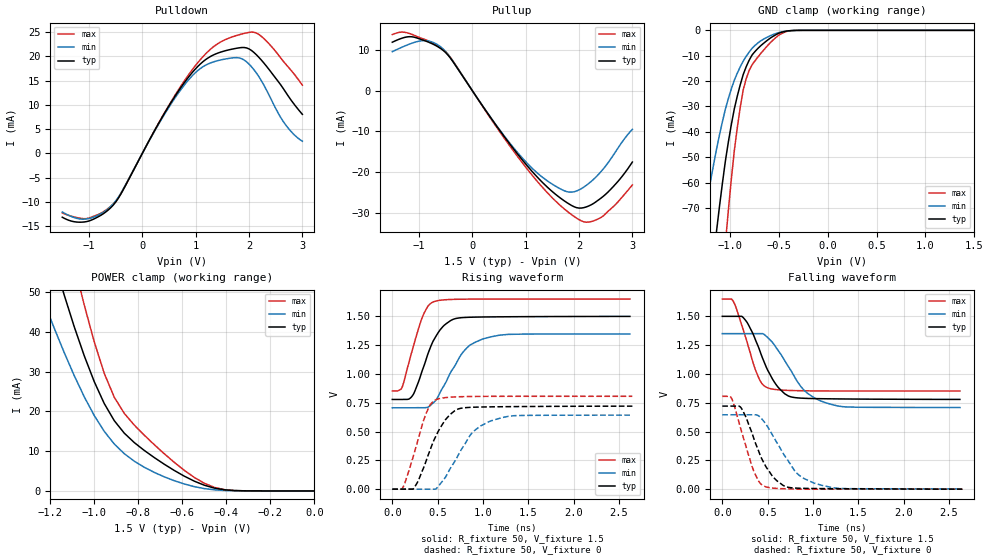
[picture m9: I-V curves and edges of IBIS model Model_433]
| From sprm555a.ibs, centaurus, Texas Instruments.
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| Model based on original model for BCSHTLTCSCDDVPBFZ_SSGFV
|   Sub model SR10_7MA_PADN_10PER_1P5
[model]   Model_433
|[Description]  [1.5V-3-STATE-X-SLOW:7MA, IND, 10%]
|   Slow slew rate (SR[1:0] = "01"), 1.14 * RExt = 0.875 * Iout
|   (I[2:0] = "010"), 7mA nominal with Rext = 50R, ,Industrial
|   temperature range (-40C to 125C, 25C nominal),10% power supply
|   tolerance
|[Input Load]
|[Output Drive] SLOW:7MA
|Voltage   1.5V
|Mode   3-STATE
Model_type   3-state
Polarity   Non-Inverting
Enable   Active-Low
Cref =  15pF
Rref =  100.0000M
Vref =  0V
Vmeas =  0.75
C_comp   1.865048p   1.676829p   1.989968p
[Temperature Range]   25   125   -40
[Voltage Range]   1.5   1.35   1.65
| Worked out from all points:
|   slope of the pulldown table from 0 to 0.225 V, typ, clamps not added: 48.9 ohm
|   slope of the pullup table from 0 to 0.225 V, typ, clamps not added: 51.5 ohm
|   GND clamp passes 1 mA (typ) near -0.49 V on its own axis
|   POWER clamp passes 1 mA (typ) near -0.47 V on its own axis
|   rising waveform, R_fixture 50, V_fixture 1.5: 20-80 % time 219ps typ, 290ps min, 176ps max; typ from 0.779 V to 1.5 V
|   rising waveform, R_fixture 50, V_fixture 0: 20-80 % time 241ps typ, 312ps min, 183ps max; typ from 0 V to 0.721 V
|   falling waveform, R_fixture 50, V_fixture 1.5: 20-80 % time 245ps typ, 333ps min, 190ps max; typ from 1.5 V to 0.779 V
|   falling waveform, R_fixture 50, V_fixture 0: 20-80 % time 242ps typ, 313ps min, 185ps max; typ from 0.721 V to 0 V
[POWER_clamp]
-1.5V     126mA      88.79mA    168.7mA
-1.242V   69.8mA     49.45mA    94.34mA
-1.136V   49.16mA    34.72mA    67.51mA
-1.061V   36.35mA    25.4mA     50.03mA
-1.045V   33.92mA    23.63mA    46.66mA
-954.5mV  21.93mA    14.95mA    29.5mA
-909.1mV  17.64mA    11.79mA    23.52mA
-863.6mV  14.51mA    9.351mA    19.47mA
-772.7mV  10.16mA    5.94mA     13.99mA
-590.9mV  3.705mA    1.741mA    5.166mA
-454.5mV  710.5uA    279.1uA    892.1uA
0V        1.424nA    14.34nA    3.127nA
[Pulldown]
-1.5V     -13.15mA   -12.08mA   -12.27mA
-1V       -13.92mA   -13.42mA   -13.31mA
-727.3mV  -12.4mA    -12.1mA    -12mA
-500mV    -10.04mA   -9.816mA   -9.874mA
272.7mV   5.543mA    5.395mA    5.589mA
681.8mV   12.92mA    12.52mA    13.17mA
1.045V    17.98mA    17.12mA    18.77mA
1.364V    20.43mA    18.95mA    22.21mA
1.818V    21.75mA    19.66mA    24.45mA
2.136V    20.34mA    16.6mA     24.8mA
2.636V    13.45mA    6.663mA    19.07mA
3V        8.041mA    2.506mA    14.06mA
[Pullup]
-1.5V     11.89mA    9.575mA    13.77mA
-1.182V   13.25mA    11.42mA    14.06mA
-954.5mV  12.56mA    12.25mA    12.88mA
-590.9mV  10.33mA    10.73mA    10.53mA
-409.1mV  7.967mA    8.059mA    8.155mA
909.1mV   -16.57mA   -16.13mA   -17.23mA
1.318V    -22.59mA   -21.31mA   -23.8mA
1.773V    -27.5mA    -24.81mA   -29.58mA
2.045V    -28.84mA   -24.06mA   -32.01mA
2.318V    -27.3mA    -21.21mA   -31.76mA
2.682V    -23mA      -15.08mA   -28.01mA
3V        -17.54mA   -9.488mA   -23.16mA
[GND_clamp]
-1.5V     -219.3mA   -131.6mA   -364.3mA
-1.288V   -134.4mA   -79.74mA   -225.6mA
-1.258V   -122.9mA   -72.77mA   -206.3mA
-1.136V   -79.27mA   -46.88mA   -132.4mA
-1.045V   -51.5mA    -31.06mA   -84.11mA
-1.015V   -44.02mA   -26.9mA    -70.91mA
-954.5mV  -31.01mA   -19.7mA    -47.55mA
-863.6mV  -17.48mA   -12.16mA   -23.55mA
-803mV    -11.81mA   -8.597mA   -15.85mA
-681.8mV  -5.986mA   -4.096mA   -9.026mA
-378.8mV  -126.2uA   -131.8uA   -179.7uA
1.5V      1.424nA    207.1nA    1.498nA
[Ramp]
dV/dt_f 0.43445765/0.24631987n 0.38788827/0.3349968n  0.4799839/0.19028011n
dV/dt_r 0.43447815/0.24147672n 0.38946568/0.3146139n 0.48494601/0.18373703n
R_load = 50
[Rising Waveform]
R_fixture = 50
V_fixture = 1.5
V_fixture_min = 1.35
V_fixture_max = 1.65
0s        778.7mV    706.2mV    852.4mV
98.8ps    778.7mV    706.2mV    868.6mV
221.7ps   810.3mV    706.2mV    1.209V
334.1ps   1.037V     706.9mV    1.498V
453ps     1.289V     749.8mV    1.625V
595.8ps   1.437V     934.8mV    1.645V
769ps     1.489V     1.178V     1.649V
992.5ps   1.494V     1.302V     1.65V
1.276ns   1.496V     1.343V     1.65V
2.62ns    1.499V     1.347V     1.65V
[Rising Waveform]
R_fixture = 50
V_fixture = 0
V_fixture_min = 0
V_fixture_max = 0
0s        0V         0V         0V
106.8ps   0V         0V         0V
234.8ps   5.638mV    0V         293.4mV
380.8ps   262.8mV    0V         671.1mV
499.4ps   490.4mV    15.82mV    781.6mV
709.4ps   690.1mV    268.9mV    801.3mV
881.3ps   710.9mV    489.6mV    804.5mV
1.088ns   714.4mV    592.9mV    805.7mV
1.395ns   716.9mV    639.4mV    806.1mV
2.647ns   720.5mV    642.4mV    806.2mV
[Falling Waveform]
R_fixture = 50
V_fixture = 1.5
V_fixture_min = 1.35
V_fixture_max = 1.65
0s        1.499V     1.349V     1.649V
115.9ps   1.499V     1.349V     1.637V
239.2ps   1.481V     1.349V     1.362V
403.1ps   1.224V     1.349V     963.7mV
500.1ps   1.033V     1.315V     879.5mV
610.8ps   888.7mV    1.209V     862.2mV
727.7ps   808.7mV    1.065V     856.6mV
903.4ps   788.3mV    856.6mV    853.4mV
1.124ns   784.3mV    753.8mV    851.9mV
2.62ns    778.5mV    708.3mV    851.4mV
[Falling Waveform]
R_fixture = 50
V_fixture = 0
V_fixture_min = 0
V_fixture_max = 0
0s        720.5mV    645.1mV    805.2mV
106.5ps   720.5mV    645.1mV    783.1mV
206.9ps   706.3mV    645.1mV    514.9mV
354.9ps   422.5mV    645.1mV    142.7mV
479ps     197.9mV    566.1mV    20.56mV
617ps     63.64mV    384.7mV    5.876mV
803.7ps   9.623mV    152.7mV    0V
1.012ns   5.701mV    52.54mV    0V
1.268ns   4.053mV    7.768mV    0V
2.647ns   0V         2.601mV    0V
